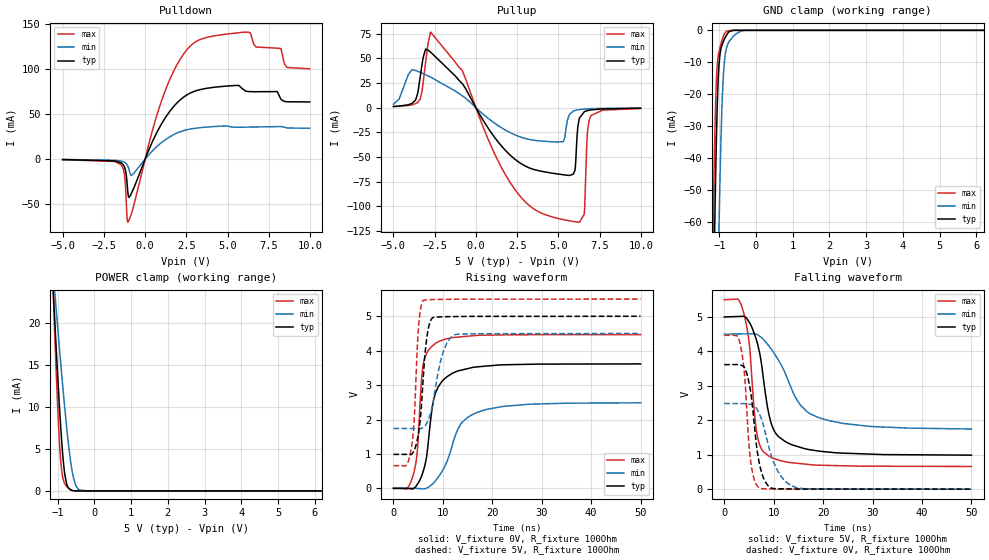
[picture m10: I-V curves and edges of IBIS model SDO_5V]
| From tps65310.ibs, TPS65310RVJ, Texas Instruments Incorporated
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[Model]   SDO_5V
Model_type   Output
Polarity   Non-Inverting
Vmeas = 2.25
Vref = 2.25
Cref = 15pF
Rref = 50
|   typ   min   max
|   (slow PVT)   (Fast PVT)   (nom PVT)
C_comp   2.616p   2.386p   2.689p
|C_comp (Hi state)   2.616p   2.386p   2.689p
|C_comp (OFF state)   2.843p   2.486p   2.854p
[Voltage Range]   5   4.5   5.5
[Temperature Range]   27   175   -40
[Pullup Reference]   5   4.5   5.5
[Pulldown Reference]   -0   -0   -0
[Power Clamp Reference]   5   4.5   5.5
[GND Clamp Reference]   -0   -0   -0
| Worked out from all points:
|   slope of the pulldown table from 0 to 0.75 V, typ, clamps not added: 24.2 ohm
|   slope of the pullup table from 0 to 0.75 V, typ, clamps not added: 36 ohm
|   GND clamp passes 1 mA (typ) near -0.77 V on its own axis
|   POWER clamp passes 1 mA (typ) near -0.76 V on its own axis
|   falling waveform, V_fixture 5V, R_fixture 100Ohm: 20-80 % time 3.04ns typ, 6.35ns min, 1.82ns max; typ from 5 V to 0.988 V
|   rising waveform, V_fixture 0V, R_fixture 100Ohm: 20-80 % time 2.44ns typ, 4.59ns min, 1.31ns max; typ from 0 V to 3.62 V
|   rising waveform, V_fixture 5V, R_fixture 100Ohm: 20-80 % time 1.33ns typ, 2.37ns min, 996ps max; typ from 0.986 V to 5 V
|   falling waveform, V_fixture 0V, R_fixture 100Ohm: 20-80 % time 1.87ns typ, 3.32ns min, 1.35ns max; typ from 3.62 V to 0 V
[Pulldown]
|   Voltage   I(typ)   I(min)   I(max)
-5V       -371.6uA   -250.6uA   -472uA
-1.46V    -3.95mA    -1.999mA   -6.002mA
-1.25V    -8.507mA   -3.314mA   -16.8mA
-1.04V    -37.57mA   -7.937mA   -69.83mA
-785mV    -36.05mA   -17.44mA   -57.79mA
1.06V     41.18mA    19.43mA    68.02mA
2.95V     75.07mA    34.13mA    128.9mA
6.28V     75.09mA    35.65mA    140.8mA
6.73V     74.9mA     35.79mA    124.5mA
8.23V     66.72mA    36.21mA    122.8mA
8.605V    63.75mA    34.66mA    101.8mA
9.985V    63.54mA    34.34mA    100.3mA
[GND Clamp]
|   Voltage   I(typ)   I(min)   I(max)
-5V       -3.827A    -3.89A     -3.808A
-1.175V   -98.93mA   -184.2mA   -67.97mA
-1.16V    -87.43mA   -172mA     -57.16mA
-1.13V    -65.69mA   -148mA     -37.82mA
-1.1V     -46.25mA   -124.9mA   -22.88mA
-1.055V   -23.59mA   -92.31mA   -10.98mA
-1.01V    -11.15mA   -63.22mA   -6.896mA
-935mV    -4.944mA   -26.84mA   -3.475mA
-890mV    -3.518mA   -14.45mA   -1.922mA
-770mV    -927.1uA   -4.363mA   -176.5uA
-320mV    0A         -32.63uA   0A
9.985V    0A         0A         0A
[Pullup]
|   Voltage   I(typ)   I(min)   I(max)
-5V       1.322mA    3.654mA    1.198mA
-3.395V   29.23mA    35.94mA    8.473mA
-2.75V    56.4mA     31.04mA    76.63mA
-830mV    24.39mA    12.12mA    37.74mA
3.16V     -60.37mA   -31.84mA   -97.91mA
5.29V     -67.83mA   -34.15mA   -113.3mA
5.905V    -67.31mA   -3.417mA   -115.1mA
6.25V     -12.22mA   -1.899mA   -115.9mA
6.565V    -4.176mA   -1.341mA   -108.1mA
6.76V     -2.921mA   -1.132mA   -25.76mA
6.985V    -2.161mA   -959.2uA   -8.054mA
9.985V    -475.2uA   -312.8uA   -726.2uA
[POWER Clamp]
|   Voltage   I(typ)   I(min)   I(max)
-5V       683.2mA    322.3mA    936.2mA
-1.13V    24.78mA    26.55mA    24.84mA
-1.07V    19.61mA    23.29mA    17.71mA
-965mV    11.13mA    17.75mA    6.919mA
-905mV    6.893mA    14.69mA    3.02mA
-860mV    4.254mA    12.47mA    1.588mA
-800mV    1.834mA    9.631mA    827.6uA
-725mV    503.6uA    6.377mA    408.9uA
-620mV    79.17uA    2.746mA    87.35uA
-500mV    5.699uA    602.6uA    3.606uA
-200mV    0A         1.19uA     0A
9.985V    0A         0A         0A
[Ramp]
R_load = 100
|   typ   min   max
dV/dt_r   2.16927/2.41962e-09   1.4912/4.51734e-09   2.67943/1.31165e-09
dV/dt_f   2.40747/3.03857e-09   1.65227/6.26486e-09   2.90476/1.82106e-09
[Falling Waveform]
V_fixture = 5V
V_fixture_min = 4.5V
V_fixture_max = 5.5V
R_fixture = 100Ohm
C_fixture = 0F
|   Time   V(typ)   V(min)   V(max)
0s        5V         4.5V       5.5V
3.813ns   5.019V     4.507V     5.179V
5.096ns   4.839V     4.51V      4.172V
6.048ns   4.522V     4.512V     2.304V
6.608ns   4.282V     4.491V     1.613V
8.772ns   2.363V     4.206V     986mV
11.16ns   1.505V     3.696V     835.4mV
15.15ns   1.225V     2.493V     745.5mV
19.1ns    1.106V     2.078V     696.2mV
50ns      987.6mV    1.746V     658.7mV
[Rising Waveform]
V_fixture = 0V
V_fixture_min = 0V
V_fixture_max = 0V
R_fixture = 100Ohm
C_fixture = 0F
|   Time   V(typ)   V(min)   V(max)
0s        1.108nV    471nV      758.9pV
2.684ns   494uV      238.1uV    -11.83mV
4.033ns   -8.221mV   357.5uV    402.8mV
4.862ns   125mV      -3.262mV   1.132V
5.542ns   305.4mV    -10.31mV   2.868V
6.048ns   509.3mV    -15.56mV   3.63V
8.505ns   2.768V     222.4mV    4.212V
13.66ns   3.432V     1.878V     4.403V
17.47ns   3.536V     2.233V     4.448V
50ns      3.615V     2.485V     4.466V
[Rising Waveform]
V_fixture = 5V
V_fixture_min = 4.5V
V_fixture_max = 5.5V
R_fixture = 100Ohm
C_fixture = 0F
|   Time   V(typ)   V(min)   V(max)
0s        986mV      1.738V     658.5mV
3.508ns   980.5mV    1.739V     1.083V
4.185ns   1.098V     1.738V     1.945V
5.096ns   1.624V     1.735V     4.713V
6.048ns   3.249V     1.768V     5.462V
6.756ns   4.389V     1.899V     5.479V
7.602ns   4.899V     2.239V     5.484V
9.914ns   4.984V     3.888V     5.491V
12.18ns   4.991V     4.447V     5.496V
50ns      5V         4.5V       5.5V
[Falling Waveform]
|Gnd
V_fixture = 0V
V_fixture_min = 0V
V_fixture_max = 0V
R_fixture = 100Ohm
C_fixture = 0F
|   Time   V(typ)   V(min)   V(max)
0s        3.616V     2.486V     4.466V
3.211ns   3.603V     2.483V     4.221V
4.033ns   3.54V      2.483V     3.425V
4.979ns   3.109V     2.472V     1.32V
5.387ns   2.777V     2.459V     759.6mV
7.069ns   769.3mV    2.198V     35.9mV
8.33ns    204.6mV    1.62V      10.21mV
10.3ns    14.32mV    674.8mV    5.478mV
14.22ns   4.468mV    64.62mV    3.57mV
50ns      17.2uV     67.06uV    4.349uV
